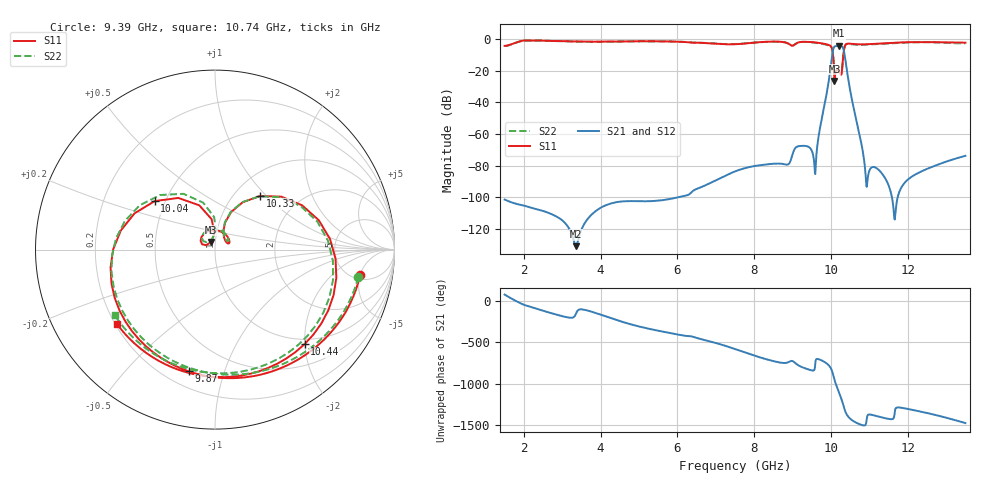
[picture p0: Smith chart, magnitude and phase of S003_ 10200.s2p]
# Hz S DB R 50
! Planar, S50180, , 20.4.1/1
! Date: 14.12.2021 19:07:46
! Data: Format (Calibration Info)
! Freq	S11:dB/Ang(--)	S21:dB/Ang(--)	S12:dB/Ang(--)	S22:dB/Ang(--)
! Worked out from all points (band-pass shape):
!   1201 points, 1.5 GHz to 13.5 GHz, reference 50 ohm
!   highest |S21| = -4.11 dB at 10.2 GHz (marker M1); lowest = -130.9 dB at 3.36 GHz (marker M2)
!   |S21| within 3 dB of the highest: 10.05 GHz to 10.33 GHz (281.6 MHz wide, 2.76 % of centre)
!   lowest |S11| = -26.4 dB at 10.09 GHz (marker M3), VSWR 1.10, Z = 47.7 + j4.09 ohm
!   |S11| at or under -10 dB: 10.05 GHz to 10.32 GHz (267.6 MHz wide, 2.63 % of centre)
!   |S22| runs from -24.4 to -0.8 dB; largest |S21 - S12| = 1.7e-06
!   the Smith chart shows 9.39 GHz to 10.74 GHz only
!   S11 on the Smith chart (normalised r, x): 9.39 GHz: 5.68, -4.99; 9.87 GHz: 0.29, -0.76; 10.04 GHz: 0.44, +0.29; 10.33 GHz: 1.31, +0.92; 10.44 GHz: 0.90, -1.99; 10.74 GHz: 0.21, -0.32
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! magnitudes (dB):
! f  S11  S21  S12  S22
! 1.5 GHz  -4.2  -101.4  -101.4  -4.3
! 3.36 GHz  -1.5  -130.9  -130.9  -1.5
! 3.5 GHz  -1.5  -120.4  -120.4  -1.5
! 5.5 GHz  -1.3  -102.0  -102.0  -1.4
! 7.5 GHz  -3.2  -83.6  -83.6  -3.1
! 8.86 GHz  -2.5  -79.3  -79.3  -2.4
! 9.1 GHz  -2.6  -68.2  -68.2  -2.6
! 9.39 GHz  -1.7  -67.8  -67.8  -1.8
! 9.5 GHz  -1.9  -70.5  -70.5  -2.0
! 9.61 GHz  -2.1  -76.5  -76.5  -2.3
! 9.87 GHz  -3.2  -36.6  -36.6  -3.5
! 9.99 GHz  -4.3  -18.2  -18.2  -4.6
! 10.04 GHz  -7.3  -8.8  -8.8  -7.3
! 10.09 GHz  -26.4  -4.7  -4.7  -24.4
! 10.2 GHz  -20.0  -4.1  -4.1  -19.8
! 10.33 GHz  -8.2  -6.8  -6.8  -8.3
! 10.44 GHz  -2.8  -23.9  -23.9  -3.0
! 10.74 GHz  -3.3  -60.0  -60.0  -3.5
! 10.93 GHz  -3.2  -93.4  -93.4  -3.4
! 11.5 GHz  -2.4  -92.4  -92.4  -2.7
! 12.69 GHz  -1.9  -80.2  -80.2  -2.0
! 13.5 GHz  -2.2  -73.7  -73.7  -2.6
